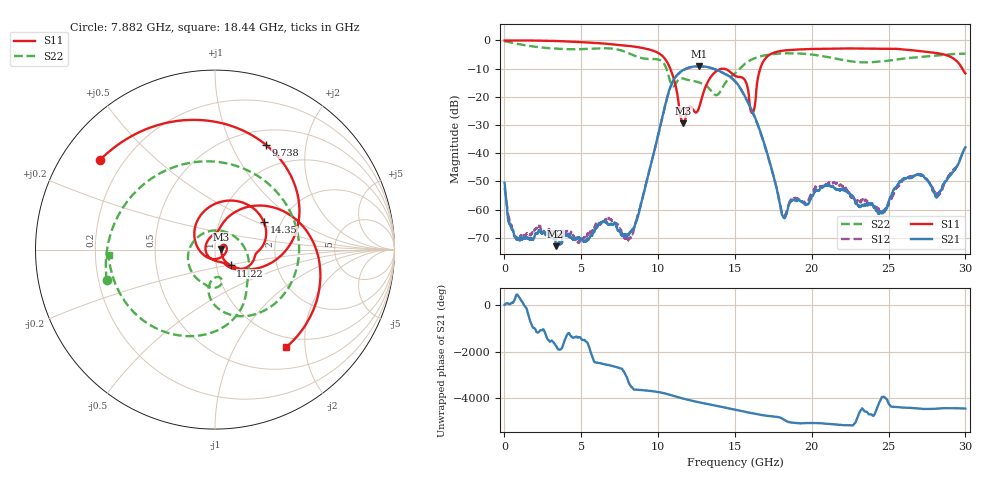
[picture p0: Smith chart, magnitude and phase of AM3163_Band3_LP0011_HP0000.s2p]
!Agilent Technologies,E8364B,MY43040894,A.07.50.67
!Agilent E8364B: A.07.50.67
!Date: Thursday, August 20, 2020 12:13:27
!Correction: S11(Full 2 Port(1,2))
!S21(Full 2 Port(1,2))
!S12(Full 2 Port(1,2))
!S22(Full 2 Port(1,2))
!S2P File: Measurements: S11, S21, S12, S22:
# Hz S  dB  R 50
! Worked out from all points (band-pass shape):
!   3201 points, 10 MHz to 30 GHz, reference 50 ohm
!   highest |S21| = -9.15 dB at 12.67 GHz (marker M1); lowest = -73.0 dB at 3.328 GHz (marker M2)
!   |S21| within 3 dB of the highest: 11.25 GHz to 14.47 GHz (3.213 GHz wide, 25 % of centre)
!   lowest |S11| = -29.4 dB at 11.65 GHz (marker M3), VSWR 1.07, Z = 53.5 + j0.348 ohm
!   |S11| at or under -10 dB: 10.79 GHz to 16.65 GHz (5.857 GHz wide, 42.7 % of centre); 29.79 GHz to end of sweep
!   |S22| runs from -19.4 to -0.3 dB; largest |S21 - S12| = 0.0045
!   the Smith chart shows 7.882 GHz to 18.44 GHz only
!   S11 on the Smith chart (normalised r, x): 7.882 GHz: 0.12, +0.34; 9.738 GHz: 0.68, +1.37; 11.22 GHz: 1.17, -0.21; 14.35 GHz: 1.63, +0.56; 18.44 GHz: 0.83, -1.65
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1e7  -0.02 -1.9  -50.51 14.8  -52.31 -44.1  -0.27 -6.5
1.143997e9  0.00 -31.4  -70.80 152.9  -69.12 -30.6  -1.53 -96.0
3.327644e9  -0.20 -90.8  -73.01 75.3  -69.37 66.2  -2.92 135.3
5.014581e9  -0.61 -135.6  -70.52 -26.6  -70.64 -149.1  -3.07 45.7
6.851469e9  -1.27 173.8  -65.15 -60.5  -63.32 -65.8  -2.82 -74.4
7.882375e9  -1.81 141.9  -68.79 -114.0  -70.03 171.3  -4.06 -164.2
8.791447e9  -2.47 108.9  -59.98 -39.4  -60.07 -32.6  -6.05 100.4
9.738006e9  -3.75 64.2  -39.52 -101.0  -39.58 -101.9  -6.58 -1.8
1.000979e10  -4.43 47.5  -33.40 -128.2  -33.50 -129.3  -6.76 -30.7
1.121876e10  -18.13 -45.2  -12.35 22.6  -12.42 22.6  -14.70 -77.8
1.164987e10  -29.39 5.5  -10.44 -53.5  -10.54 -53.6  -13.54 -98.6
1.26714e10  -23.78 -144.6  -9.15 151.2  -9.20 151.5  -14.91 -136.1
1.434897e10  -10.09 29.4  -11.80 -72.1  -11.90 -71.9  -15.28 -1.7
1.5005e10  -12.53 -3.4  -14.42 -163.1  -14.53 -163.0  -11.70 -46.6
1.6139e10  -25.73 -162.6  -25.18 40.9  -25.44 41.2  -6.63 -93.2
1.686063e10  -7.33 30.7  -35.74 -45.7  -36.07 -43.3  -5.39 -121.6
1.844448e10  -3.43 -54.0  -59.71 37.9  -59.20 43.1  -4.54 -176.9
2.000958e10  -3.01 -100.2  -55.27 -14.6  -53.70 -17.1  -4.99 127.5
2.255873e10  -2.84 -159.1  -55.04 -115.7  -55.61 -120.3  -7.44 13.4
2.500479e10  -3.01 144.1  -57.23 92.9  -57.53 -116.4  -7.17 -100.7
2.818186e10  -4.52 53.2  -55.35 -115.6  -54.46 -114.2  -5.28 151.5
3e10  -11.69 -28.9  -37.90 -117.1  -38.06 -114.4  -4.69 99.1
